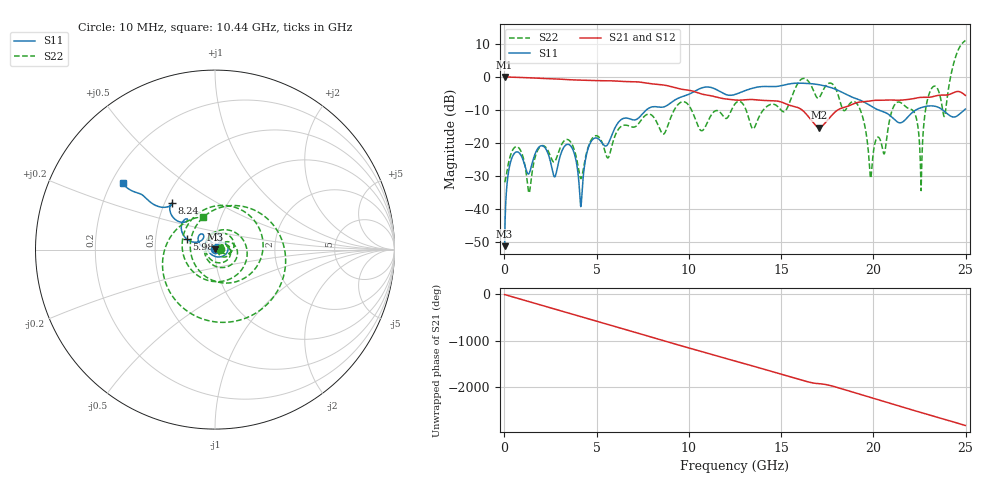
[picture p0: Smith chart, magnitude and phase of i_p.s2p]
!Keysight Technologies,N5245B,MY57181346,A.12.70.07
!Automatic Fixture Removal (AFR)
!Date: Wednesday, November 07, 2018 11:53:30 AM
!S2P File: Measurements: S11,S21,S12,S22:
# MHz S  RI  R 50
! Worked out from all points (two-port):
!   2499 points, 10 MHz to 24.99 GHz, reference 50 ohm
!   highest |S21| = 0.00 dB at 10 MHz (marker M1); lowest = -15.4 dB at 17.07 GHz (marker M2)
!   |S21| within 3 dB of the highest: start of sweep to 9.077 GHz
!   lowest |S11| = -51.3 dB at 10 MHz (marker M3), VSWR 1.01, Z = 50.2 + j0.168 ohm
!   |S11| at or under -10 dB: start of sweep to 7.695 GHz; 20.27 GHz to 22.31 GHz (2.038 GHz wide, 9.57 % of centre); 23.76 GHz to 24.94 GHz (1.18 GHz wide, 4.85 % of centre)
!   |S22| runs from -35.1 to 11.0 dB; largest |S21 - S12| = 1.4e-15
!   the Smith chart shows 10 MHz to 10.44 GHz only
!   S11 on the Smith chart (normalised r, x): 10 MHz: 1.00, +0.00; 5.98 GHz: 0.73, +0.09; 8.24 GHz: 0.55, +0.33; 10.44 GHz: 0.25, +0.30
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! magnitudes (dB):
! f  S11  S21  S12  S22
! 10 MHz  -51.3  0.0  0.0  -31.9
! 630 MHz  -22.8  -0.1  -0.1  -21.1
! 1.34 GHz  -29.2  -0.3  -0.3  -35.1
! 3.52 GHz  -20.6  -0.9  -0.9  -19.3
! 4.18 GHz  -37.3  -1.0  -1.0  -30.6
! 4.67 GHz  -19.8  -1.1  -1.1  -19.5
! 5.98 GHz  -15.6  -1.2  -1.2  -18.1
! 8.24 GHz  -9.0  -2.2  -2.2  -13.5
! 8.34 GHz  -9.1  -2.3  -2.3  -14.7
! 10.44 GHz  -4.0  -4.7  -4.7  -14.2
! 12.5 GHz  -5.3  -7.0  -7.0  -8.2
! 13.5 GHz  -3.4  -6.9  -6.9  -15.7
! 16.67 GHz  -2.1  -13.3  -13.3  -3.1
! 17.07 GHz  -2.4  -15.4  -15.4  -6.3
! 19.12 GHz  -6.7  -7.8  -7.8  -8.2
! 19.86 GHz  -8.8  -7.2  -7.2  -30.7
! 20.83 GHz  -11.4  -7.0  -7.0  -14.5
! 22.11 GHz  -10.8  -6.7  -6.7  -10.0
! 22.59 GHz  -9.3  -6.2  -6.2  -34.4
! 23.06 GHz  -8.8  -6.2  -6.2  -4.6
! 23.86 GHz  -10.5  -5.5  -5.5  -11.9
! 24.99 GHz  -9.8  -5.6  -5.6  11.0
